FUNCTION FC 10 : VOID
TITLE =COMANDI PROFIBUS AZIONAMENTO 10 PROFILA 8 (SLAVE 7)
VERSION : 0.1

BEGIN
NETWORK
TITLE =TRASFERISCO I SEGNALI DI COMANDO
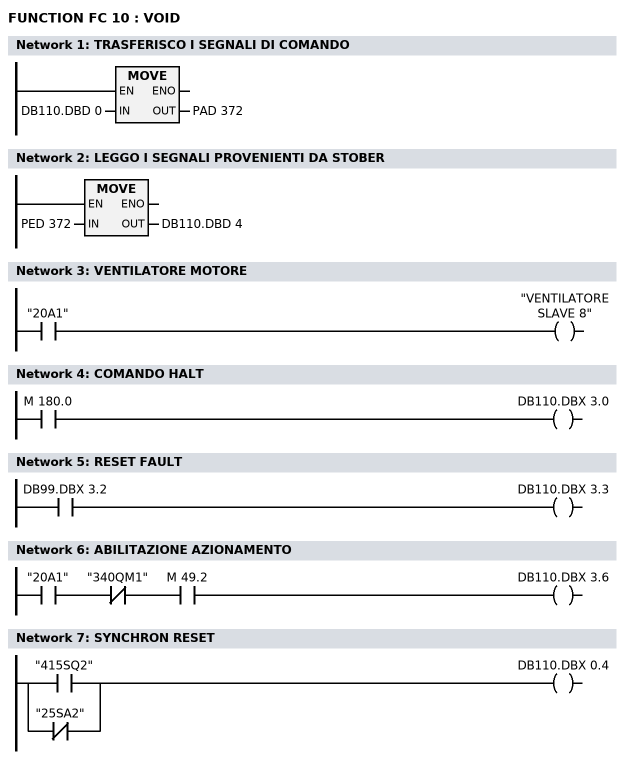
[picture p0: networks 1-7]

      L     DB110.DBD    0;
      T     PAD  372;
      NOP   0;
NETWORK
TITLE =LEGGO I SEGNALI PROVENIENTI DA STOBER

      L     PED  372;
      T     DB110.DBD    4;
      NOP   0;
NETWORK
TITLE =VENTILATORE MOTORE

      U     "20A1";
      =     "VENTILATORE SLAVE 8";
NETWORK
TITLE =COMANDO HALT

      U     M    180.0;
      =     DB110.DBX    3.0;
NETWORK
TITLE =RESET FAULT

      U     DB99.DBX    3.2;
      =     DB110.DBX    3.3;
NETWORK
TITLE =ABILITAZIONE AZIONAMENTO

      U     "20A1";
      UN    "340QM1";
      U     M     49.2;
      =     DB110.DBX    3.6;
NETWORK
TITLE =SYNCHRON RESET

      O     "415SQ2";
      ON    "25SA2";
      =     DB110.DBX    0.4;
END_FUNCTION

